(* Logix 5000 AddOnInstructionDefinition export AMCI_NXFE2_Jog_CW; software revision 20.03 *)

ADD_ON_INSTRUCTION AMCI_NXFE2_Jog_CW   (* revision 1.0, vendor AMCI, ExecuteEnableInFalse *)
VAR_INPUT
   Axis_Status_Bits : INT; {required}
   _0_normal_1_S_Curve_Acceleration : BOOL;
   _0_Triangular_1_Trapezoidal_S_Curve : BOOL;
   Programmed_Speed : DINT; {required}
   Acceleration : INT; {required}
   Deceleration : INT; {required}
END_VAR
VAR_IN_OUT
   NXFE2_output_data : _000A:NXFE2_0986AEB4:O:0; {required}
END_VAR
VAR_OUTPUT
   EN : BOOL; {access Read Only, visible}
   Jog_CW_Occurring : BOOL; {access Read Only, visible}
   ER : BOOL; {access Read Only, visible}
END_VAR
VAR
   command_data_block : INT[10];
        [0]   // Command Bits MSW
        [1]   // Command Bits LSW
        [3]   // Lower Target Position
        [4]   // Upper Programmed Speed
        [5]   // Lower Programmed Speed
END_VAR

ROUTINE EnableInFalse   (* ladder *)
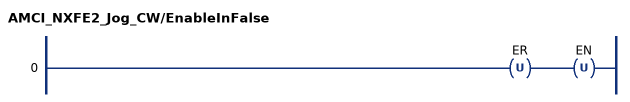
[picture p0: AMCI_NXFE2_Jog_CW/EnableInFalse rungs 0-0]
   0: OTU(ER)OTU(EN);
END_ROUTINE

ROUTINE Logic   (* ladder *)
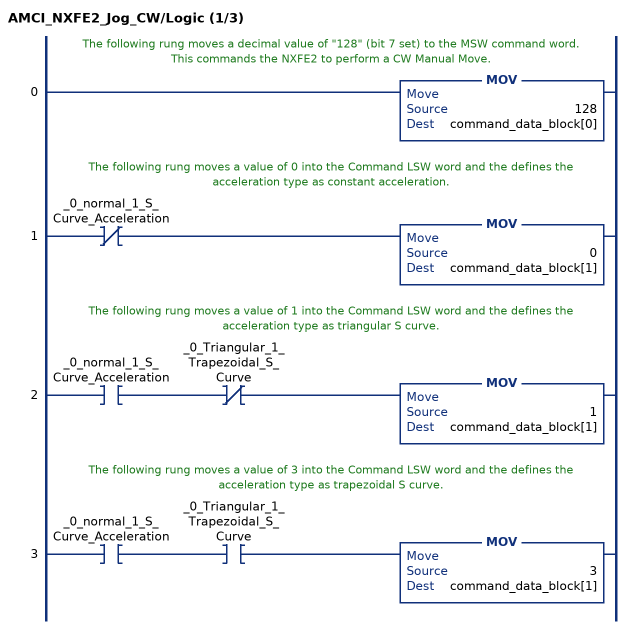
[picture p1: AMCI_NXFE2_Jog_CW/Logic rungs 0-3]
   // The following rung moves a decimal value of "128" (bit 7 set) to the MSW command word.  This commands the NXFE2 to perform a CW Manual Move.
   0: MOV(128,command_data_block[0]);
   // The following rung moves a value of 0 into the Command LSW word and the defines the acceleration type as constant acceleration.
   1: XIO(_0_normal_1_S_Curve_Acceleration)MOV(0,command_data_block[1]);
   // The following rung moves a value of 1 into the Command LSW word and the defines the acceleration type as triangular S curve.
   2: XIC(_0_normal_1_S_Curve_Acceleration)XIO(_0_Triangular_1_Trapezoidal_S_Curve)MOV(1,command_data_block[1]);
   // The following rung moves a value of 3 into the Command LSW word and the defines the acceleration type as trapezoidal S curve.
   3: XIC(_0_normal_1_S_Curve_Acceleration)XIC(_0_Triangular_1_Trapezoidal_S_Curve)MOV(3,command_data_block[1]);
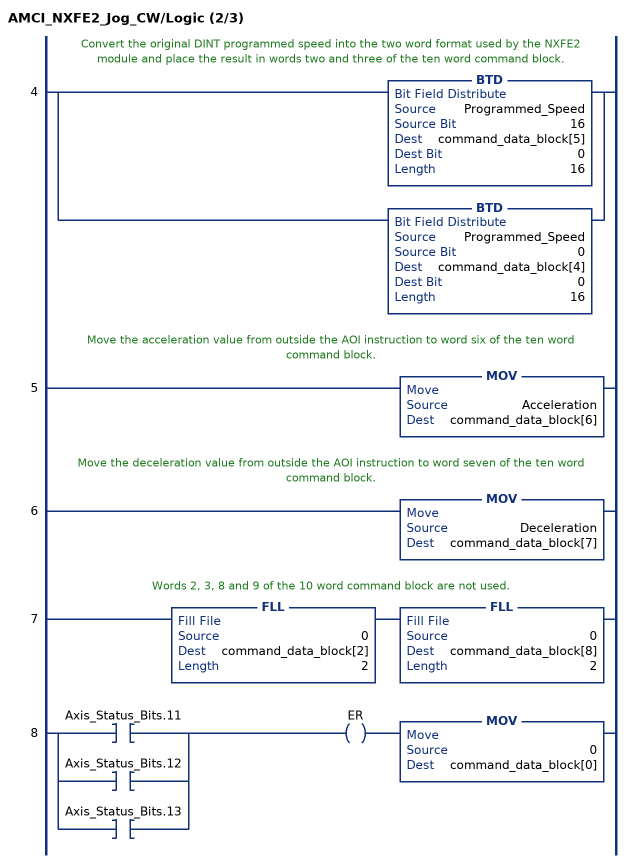
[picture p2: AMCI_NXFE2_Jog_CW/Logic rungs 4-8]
   // Convert the original DINT programmed speed into the two word format used by the NXFE2 module and place the result in words two and three of the ten word command block.
   4: [BTD(Programmed_Speed,16,command_data_block[5],0,16) ,BTD(Programmed_Speed,0,command_data_block[4],0,16) ];
   // Move the acceleration value from outside the AOI instruction to word six of the ten word command block.
   5: MOV(Acceleration,command_data_block[6]);
   // Move the deceleration value from outside the AOI instruction to word seven of the ten word command block.
   6: MOV(Deceleration,command_data_block[7]);
   // Words 2, 3, 8 and 9 of the 10 word command block are not used.
   7: FLL(0,command_data_block[2],2)FLL(0,command_data_block[8],2);
   8: [XIC(Axis_Status_Bits.11) ,XIC(Axis_Status_Bits.12) ,XIC(Axis_Status_Bits.13) ]OTE(ER)MOV(0,command_data_block[0]);
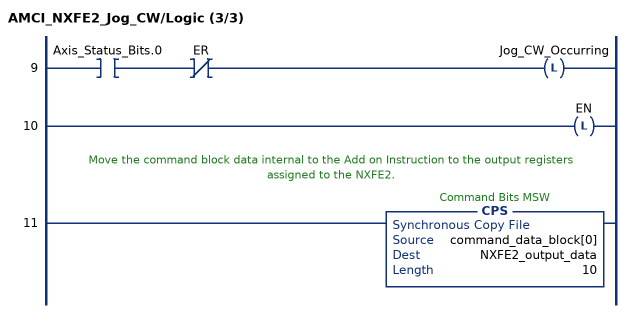
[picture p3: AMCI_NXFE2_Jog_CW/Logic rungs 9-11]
   9: XIC(Axis_Status_Bits.0)XIO(ER)OTL(Jog_CW_Occurring);
   10: OTL(EN);
   // Move the command block data internal to the Add on Instruction to the output registers assigned to the NXFE2.
   11: CPS(command_data_block[0],NXFE2_output_data,10);
END_ROUTINE
END_ADD_ON_INSTRUCTION
